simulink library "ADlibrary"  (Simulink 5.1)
undefined symbols (not defined in the file or in its folder): fifo_length, MCLK
libraries: xbsIndex_r3 x112, ADlibrary x9, xrbsControl_r3 x3

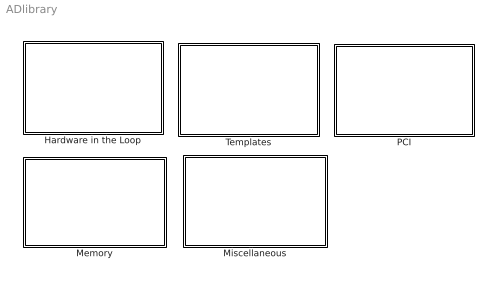
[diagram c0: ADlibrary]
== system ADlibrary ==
  Hardware in the Loop : Subsystem
  Memory : Subsystem
  Miscellaneous : Subsystem
  PCI : Subsystem
  Templates : Subsystem

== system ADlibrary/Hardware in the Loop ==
  ADMXRC DWSR IO : S-Function  AncestorBlock=ADlibrary/ADMXRC SWDR I//O  FunctionName=ADMXRCdwsr  Parameters=filename clock_freq mclk_freq input_width output_width index  mask(ADMXRC DWSR I/O){filename=, clock_freq=50, mclk_freq=, input_width=1, output_width=1, index=0}
      mask prompts: clock_freq "L Clock Frequency (MHz)"; mclk_freq "M Clock Frequency (MHz) (x2 for XRC-II)"; input_width "Width of input vector"; output_width "Width of output vector"; index "Card Index"
      mask help: Hardware in the loop block for Demand Mode DMA Write, Slave mode Read I/O with ADM-XRC/ADM-XRC II Cards.
      mask init:
      | try
      | card=admxrc_init([],index);
      | [id,sn,bt,ft]=admxrc_getinfo(card);
      | admxrc_close(card);
      | infostr=['Board Type: ' bt ' - FPGA : ' ft];
      | catch
      | infostr='No Card Detected';
      | end
      | 
      | pos=get_param(gcb,'Position');
      | width=pos(3)-pos(1);
      | height=pos(4)-pos(2);
      | if (input_width>0),istr=['Input [' num2str(input_width) ']'];else,istr='';end
      | if (output_width>0), ostr=['Output [' num2str(output_width) ']'];else,ostr='';end
      | as=get_param(gcb,'MaskIconUnits');
      | if (as(1)=='p')
      | 	im=imread('adbutton.jpg');s=get_param(gcb,'MaskDisplay');
      |     add_ad_icon(70,15);
      | else	
      | 	rm_ad_icon
      | end
  ADMXRC MMAP IO : S-Function  FunctionName=ADMXRCmmap  Parameters=filename clock_freq mclk_freq index  mask(ADMXRC MMAP I/O){filename=, clock_freq=50, mclk_freq=25, index=0}
      mask prompts: clock_freq "L Clock Frequency (MHz)"; mclk_freq "M Clock Frequency (MHz) (x2 for XRC-II)"; index "Card Index"
      mask help: Hardware in the loop block for Memory Mapped I/O Communication with ADM-XRC/ADM-XRC II Cards.
      mask init:
      | try
      | card=admxrc_init([],index);
      | [id,sn,bt,ft]=admxrc_getinfo(card);
      | admxrc_close(card);
      | infostr=['Board: ' bt ' - FPGA : ' ft];
      | catch
      | infostr='No Card Detected';
      | end
      | 
      | pos=get_param(gcb,'Position');
      | width=pos(3)-pos(1);
      | height=pos(4)-pos(2);
      | as=get_param(gcb,'MaskIconUnits');
      | if (as(1)=='p')
      | 	im=imread('adbutton.jpg');s=get_param(gcb,'MaskDisplay');
      |     add_ad_icon(70,15);
      | else	
      | 	rm_ad_icon
      | end
  ADMXRC SWDR IO : S-Function  AncestorBlock=ADlibrary/ADMXRC Slave I//O  FunctionName=ADMXRCswdr  Parameters=filename clock_freq mclk_freq input_width output_width index  mask(ADMXRC SWDR I/O){filename=, clock_freq=50, mclk_freq=, input_width=1, output_width=1, index=0}
      mask prompts: clock_freq "L Clock Frequency (MHz)"; mclk_freq "M Clock Frequency (MHz) (x2 for XRC-II)"; input_width "Width of input vector"; output_width "Width of output vector"; index "Card Index"
      mask help: Hardware in the loop block for Slave Mode Write, Demand Mode DMA Read to ADM-XRC/ADM-XRC II Cards.
      mask init:
      | try
      | card=admxrc_init([],index);
      | [id,sn,bt,ft]=admxrc_getinfo(card);
      | admxrc_close(card);
      | infostr=['Board Type: ' bt ' - FPGA : ' ft];
      | catch
      | infostr='No Card Detected';
      | end
      | 
      | pos=get_param(gcb,'Position');
      | width=pos(3)-pos(1);
      | height=pos(4)-pos(2);
      | if (input_width>0),istr=['Input [' num2str(input_width) ']'];else,istr='';end
      | if (output_width>0), ostr=['Output [' num2str(output_width) ']'];else,ostr='';end
      | as=get_param(gcb,'MaskIconUnits');
      | if (as(1)=='p')
      | 	im=imread('adbutton.jpg');s=get_param(gcb,'MaskDisplay');
      |     add_ad_icon(70,15);
      | else	
      | 	rm_ad_icon
      | end
  ADMXRC Slave IO : S-Function  AncestorBlock=ADlibrary/ADMXRC Simple I//O  FunctionName=ADMXRCslave  Parameters=filename clock_freq input_width output_width tll index  mask(ADMXRC Slave I/O){filename=, clock_freq=50, input_width=1, output_width=1, tll=1000, index=0}
      mask prompts: clock_freq "L Clock Frequency (MHz)"; input_width "Width of input vector"; output_width "Width of output vector"; tll "Terminate Loop Limit"; index "Card Index"
      mask help: Hardware in the loop block for Slave Mode Access to ADM-XRC/ADM-XRC II Cards.
      mask init:
      | try
      | card=admxrc_init([],index);
      | [id,sn,bt,ft]=admxrc_getinfo(card);
      | admxrc_close(card);
      | infostr=['Board Type: ' bt ' - FPGA : ' ft];
      | catch
      | infostr='No Card Detected';
      | end
      | 
      | pos=get_param(gcb,'Position');
      | width=pos(3)-pos(1);
      | height=pos(4)-pos(2);
      | if (input_width>0),istr=['Input [' num2str(input_width) ']'];else,istr='';end
      | if (output_width>0), ostr=['Output [' num2str(output_width) ']'];else,ostr='';end
      | as=get_param(gcb,'MaskIconUnits');
      | if (as(1)=='p')
      | 	im=imread('adbutton.jpg');s=get_param(gcb,'MaskDisplay');
      |     add_ad_icon(70,15);
      | else	
      | 	rm_ad_icon
      | end

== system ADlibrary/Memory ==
  XRCSRAM0 : Subsystem
  XRCSRAM1 : Subsystem  AncestorBlock=ADlibrary/SRAM0
  XRCSRAM2 : Subsystem  AncestorBlock=ADlibrary/SRAM0
  XRCSRAM3 : Subsystem  AncestorBlock=ADlibrary/SRAM0
  XRCSRAM4 : Subsystem  AncestorBlock=ADlibrary/SRAM0
  XRCSRAM5 : Subsystem  AncestorBlock=ADlibrary/SRAM0
  XRCSRAM7 : Subsystem

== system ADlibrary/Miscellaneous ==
  ADMXRC Board  Implementation : Subsystem  mask(Board Implementation){board=<empty>, run_synth=off, make_clean=off, userdefmods=, custom_template_file=, lvds_io_std=3.3v, clock_source=MCLK, mclk_pin=}
      mask prompts: run_synth "Run Synthesis"; make_clean "Make Clean"; userdefmods "User Defined I/O Modules"; custom_template_file "Custom Template File"; lvds_io_std "LVDS I/O Standard"; clock_source "Clock Source"; mclk_pin "MCLK Pin"
      mask help: This block allows the implementation of the system on an FPGA situated on an XRC board. This modifies the system generator VHDL and adds extra code to connect to the PCI bus, and support the ZBT SRAM and XRC I/O ports. The block can also autorun Xilinx and Third Party Synthesis tools.
      mask init:
      | as=get_param(gcb,'MaskIconUnits');
      | if (as(1)=='p')
      | 	im=imread('adbutton.jpg');s=get_param(gcb,'MaskDisplay');
      |     add_ad_icon(14,3);
      | else	
      | 	rm_ad_icon
      | end
  Complex  to int32 : S-Function  FunctionName=cplxtoint32
  HEX Constant : Subsystem  mask(HEX Constant){value=1234}
      mask prompts: value "HEX Constant"
      mask help: Hexadecimal constant
  HEX Display : S-Function  FunctionName=hexdisplay
  XRC Scope : Subsystem
  int32 to Complex : S-Function  FunctionName=int32tocplx

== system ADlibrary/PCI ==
  DWSR XRCPCI : Subsystem  AncestorBlock=ADlibrary/PCI/Slave XRCPCI  mask{no_inputs=1, no_outputs=1, circuit_lag=1, decode_delay=0}
      mask prompts: no_inputs "Number of Inputs"; no_outputs "Number of Outputs"; circuit_lag "Circuit Lag"; decode_delay "Decode Delay"
      mask init:
      | pos=get_param(gcb,'Position');
      | width=pos(3)-pos(1);height=pos(4)-pos(2);
      | if (no_inputs>0),istr=['Input [' num2str(no_inputs) ']'];else,istr='';end
      | if (no_outputs>0), ostr=['Output [' num2str(no_outputs) ']'];else,ostr='';end
      | as=get_param(gcb,'MaskIconUnits');
      | if (as(1)=='p')
      | 	im=imread('adbutton.jpg');s=get_param(gcb,'MaskDisplay');
      |     add_ad_icon(60,80);
      | else	
      | 	rm_ad_icon
      | end
  MMAP XRCPCI : Subsystem  AncestorBlock=ADlibrary/PCI/DWSR XRCPCI  mask(MMAP XRCPCI){qv132678sdfs=0}
      mask prompts: qv132678sdfs "a"
      mask init:
      | pos=get_param(gcb,'Position');
      | width=pos(3)-pos(1);height=pos(4)-pos(2);
      | as=get_param(gcb,'MaskIconUnits');
      | if (as(1)=='p')
      | 	im=imread('adbutton.jpg');s=get_param(gcb,'MaskDisplay');
      |     add_ad_icon(60,80);
      | else	
      | 	rm_ad_icon
      | end
  SWDR XRCPCI : Subsystem  AncestorBlock=ADlibrary/PCI/ADMA XRCPCI  mask{no_inputs=1, no_outputs=1, circuit_lag=4, fifo_length=256, debug=0}
      mask prompts: no_inputs "Number of Inputs"; no_outputs "Number of Outputs"; circuit_lag "Circuit Lag"; fifo_length "FIFO Length"; debug "Debug Flag"
      mask init:
      | pos=get_param(gcb,'Position');
      | width=pos(3)-pos(1);height=pos(4)-pos(2);
      | if (no_inputs>0),istr=['Input [' num2str(no_inputs) ']'];else,istr='';end
      | if (no_outputs>0), ostr=['Output [' num2str(no_outputs) ']'];else,ostr='';end
      | as=get_param(gcb,'MaskIconUnits');
      | if (as(1)=='p')
      | 	im=imread('adbutton.jpg');s=get_param(gcb,'MaskDisplay');
      |     add_ad_icon(60,80);
      | else	
      | 	rm_ad_icon
      | end
  Slave XRCPCI : Subsystem  mask{no_inputs=1, no_outputs=1, circuit_lag=1, decode_delay=0}
      mask prompts: no_inputs "Number of Inputs"; no_outputs "Number of Outputs"; circuit_lag "Circuit Lag"; decode_delay "Decode Delay"
      mask init:
      | pos=get_param(gcb,'Position');
      | width=pos(3)-pos(1);height=pos(4)-pos(2);
      | if (no_inputs>0),istr=['Input [' num2str(no_inputs) ']'];else,istr='';end
      | if (no_outputs>0), ostr=['Output [' num2str(no_outputs) ']'];else,ostr='';end
      | as=get_param(gcb,'MaskIconUnits');
      | if (as(1)=='p')
      | 	im=imread('adbutton.jpg');s=get_param(gcb,'MaskDisplay');
      |     add_ad_icon(60,80);
      | else	
      | 	rm_ad_icon
      | end

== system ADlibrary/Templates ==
  DWSR IO : Subsystem
  MMAP IO : Subsystem  AncestorBlock=ADlibrary/Templates/DWSR IO
  SWDR IO : Subsystem
  SlaveIO : Subsystem

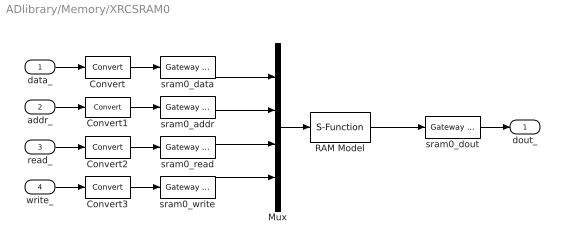
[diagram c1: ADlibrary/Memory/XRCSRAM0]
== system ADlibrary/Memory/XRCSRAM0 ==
  data_ : Inport
  addr_ : Inport  Port=2
  read_ : Inport  Port=3
  write_ : Inport  Port=4
  Convert : xbsIndex_r3/Convert  arith_type="Signed  (2's comp)"  n_bits=32  bin_pt=0  quantization=Truncate  overflow=Wrap  latency=0  explicit_period=off  period=1  dbl_ovrd=off  inserted_by_tool=off
  Convert1 : xbsIndex_r3/Convert  arith_type=Unsigned  n_bits=20  bin_pt=0  quantization=Truncate  overflow=Wrap  latency=0  explicit_period=off  period=1  dbl_ovrd=off  inserted_by_tool=off
  Convert2 : xbsIndex_r3/Convert  arith_type=Boolean  n_bits=1  bin_pt=0  quantization=Truncate  overflow=Wrap  latency=0  explicit_period=off  period=1  dbl_ovrd=off  inserted_by_tool=off
  Convert3 : xbsIndex_r3/Convert  arith_type=Boolean  n_bits=1  bin_pt=0  quantization=Truncate  overflow=Wrap  latency=0  explicit_period=off  period=1  dbl_ovrd=off  inserted_by_tool=off
  Mux : Mux
  RAM Model : S-Function  FunctionName=modelram  Parameters=0
  sram0_addr : xbsIndex_r3/Gateway Out  hdl_port=on  timing_constraint=None  locs_specified=off  LOCs={}  needs_fixed_name=on
  sram0_data : xbsIndex_r3/Gateway Out  hdl_port=on  timing_constraint=None  locs_specified=off  LOCs={}  needs_fixed_name=on
  sram0_dout : xbsIndex_r3/Gateway In  arith_type="Signed  (2's comp)"  n_bits=32  bin_pt=0  quantization=Truncate  overflow=Wrap  period=1  timing_constraint=None  locs_specified=off  LOCs={}  needs_fixed_name=on  dbl_ovrd=off
  sram0_read : xbsIndex_r3/Gateway Out  hdl_port=on  timing_constraint=None  locs_specified=off  LOCs={}  needs_fixed_name=on
  sram0_write : xbsIndex_r3/Gateway Out  hdl_port=on  timing_constraint=None  locs_specified=off  LOCs={}  needs_fixed_name=on
  dout_ : Outport
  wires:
  data_/1 -> Convert/1
  addr_/1 -> Convert1/1
  read_/1 -> Convert2/1
  sram0_dout/1 -> dout_/1
  Convert/1 -> sram0_data/1
  Convert1/1 -> sram0_addr/1
  Convert2/1 -> sram0_read/1
  RAM Model/1 -> sram0_dout/1
  Mux/1 -> RAM Model/1
  sram0_data/1 -> Mux/1
  sram0_addr/1 -> Mux/2
  sram0_read/1 -> Mux/3
  write_/1 -> Convert3/1
  Convert3/1 -> sram0_write/1
  sram0_write/1 -> Mux/4

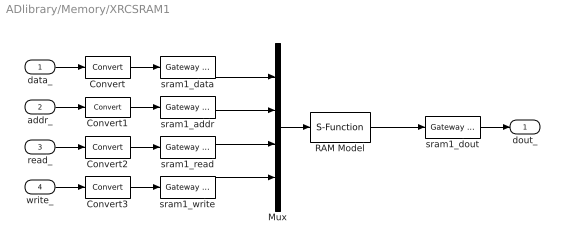
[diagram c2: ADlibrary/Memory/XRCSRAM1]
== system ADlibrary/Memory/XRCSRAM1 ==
  data_ : Inport
  addr_ : Inport  Port=2
  read_ : Inport  Port=3
  write_ : Inport  Port=4
  Convert : xbsIndex_r3/Convert  arith_type="Signed  (2's comp)"  n_bits=32  bin_pt=0  quantization=Truncate  overflow=Wrap  latency=0  explicit_period=off  period=1  dbl_ovrd=off  inserted_by_tool=off
  Convert1 : xbsIndex_r3/Convert  arith_type=Unsigned  n_bits=20  bin_pt=0  quantization=Truncate  overflow=Wrap  latency=0  explicit_period=off  period=1  dbl_ovrd=off  inserted_by_tool=off
  Convert2 : xbsIndex_r3/Convert  arith_type=Boolean  n_bits=1  bin_pt=0  quantization=Truncate  overflow=Wrap  latency=0  explicit_period=off  period=1  dbl_ovrd=off  inserted_by_tool=off
  Convert3 : xbsIndex_r3/Convert  arith_type=Boolean  n_bits=1  bin_pt=0  quantization=Truncate  overflow=Wrap  latency=0  explicit_period=off  period=1  dbl_ovrd=off  inserted_by_tool=off
  Mux : Mux
  RAM Model : S-Function  FunctionName=modelram  Parameters=1
  sram1_addr : xbsIndex_r3/Gateway Out  hdl_port=on  timing_constraint=None  locs_specified=off  LOCs={}  needs_fixed_name=on
  sram1_data : xbsIndex_r3/Gateway Out  hdl_port=on  timing_constraint=None  locs_specified=off  LOCs={}  needs_fixed_name=on
  sram1_dout : xbsIndex_r3/Gateway In  arith_type="Signed  (2's comp)"  n_bits=32  bin_pt=0  quantization=Truncate  overflow=Wrap  period=1  timing_constraint=None  locs_specified=off  LOCs={}  needs_fixed_name=on  dbl_ovrd=off
  sram1_read : xbsIndex_r3/Gateway Out  hdl_port=on  timing_constraint=None  locs_specified=off  LOCs={}  needs_fixed_name=on
  sram1_write : xbsIndex_r3/Gateway Out  hdl_port=on  timing_constraint=None  locs_specified=off  LOCs={}  needs_fixed_name=on
  dout_ : Outport
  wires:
  sram1_write/1 -> Mux/4
  Convert3/1 -> sram1_write/1
  write_/1 -> Convert3/1
  sram1_read/1 -> Mux/3
  sram1_addr/1 -> Mux/2
  sram1_data/1 -> Mux/1
  Mux/1 -> RAM Model/1
  RAM Model/1 -> sram1_dout/1
  Convert2/1 -> sram1_read/1
  Convert1/1 -> sram1_addr/1
  Convert/1 -> sram1_data/1
  sram1_dout/1 -> dout_/1
  read_/1 -> Convert2/1
  addr_/1 -> Convert1/1
  data_/1 -> Convert/1

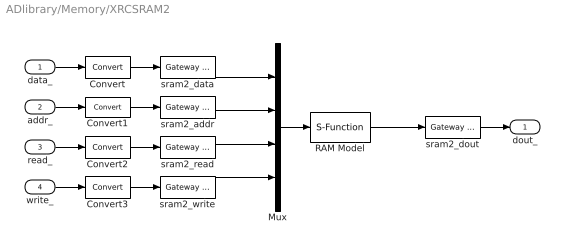
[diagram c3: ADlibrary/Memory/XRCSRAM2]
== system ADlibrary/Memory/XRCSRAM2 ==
  data_ : Inport
  addr_ : Inport  Port=2
  read_ : Inport  Port=3
  write_ : Inport  Port=4
  Convert : xbsIndex_r3/Convert  arith_type="Signed  (2's comp)"  n_bits=32  bin_pt=0  quantization=Truncate  overflow=Wrap  latency=0  explicit_period=off  period=1  dbl_ovrd=off  inserted_by_tool=off
  Convert1 : xbsIndex_r3/Convert  arith_type=Unsigned  n_bits=20  bin_pt=0  quantization=Truncate  overflow=Wrap  latency=0  explicit_period=off  period=1  dbl_ovrd=off  inserted_by_tool=off
  Convert2 : xbsIndex_r3/Convert  arith_type=Boolean  n_bits=1  bin_pt=0  quantization=Truncate  overflow=Wrap  latency=0  explicit_period=off  period=1  dbl_ovrd=off  inserted_by_tool=off
  Convert3 : xbsIndex_r3/Convert  arith_type=Boolean  n_bits=1  bin_pt=0  quantization=Truncate  overflow=Wrap  latency=0  explicit_period=off  period=1  dbl_ovrd=off  inserted_by_tool=off
  Mux : Mux
  RAM Model : S-Function  FunctionName=modelram  Parameters=2
  sram2_addr : xbsIndex_r3/Gateway Out  hdl_port=on  timing_constraint=None  locs_specified=off  LOCs={}  needs_fixed_name=on
  sram2_data : xbsIndex_r3/Gateway Out  hdl_port=on  timing_constraint=None  locs_specified=off  LOCs={}  needs_fixed_name=on
  sram2_dout : xbsIndex_r3/Gateway In  arith_type="Signed  (2's comp)"  n_bits=32  bin_pt=0  quantization=Truncate  overflow=Wrap  period=1  timing_constraint=None  locs_specified=off  LOCs={}  needs_fixed_name=on  dbl_ovrd=off
  sram2_read : xbsIndex_r3/Gateway Out  hdl_port=on  timing_constraint=None  locs_specified=off  LOCs={}  needs_fixed_name=on
  sram2_write : xbsIndex_r3/Gateway Out  hdl_port=on  timing_constraint=None  locs_specified=off  LOCs={}  needs_fixed_name=on
  dout_ : Outport
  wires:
  sram2_write/1 -> Mux/4
  Convert3/1 -> sram2_write/1
  write_/1 -> Convert3/1
  sram2_read/1 -> Mux/3
  sram2_addr/1 -> Mux/2
  sram2_data/1 -> Mux/1
  Mux/1 -> RAM Model/1
  RAM Model/1 -> sram2_dout/1
  Convert2/1 -> sram2_read/1
  Convert1/1 -> sram2_addr/1
  Convert/1 -> sram2_data/1
  sram2_dout/1 -> dout_/1
  read_/1 -> Convert2/1
  addr_/1 -> Convert1/1
  data_/1 -> Convert/1

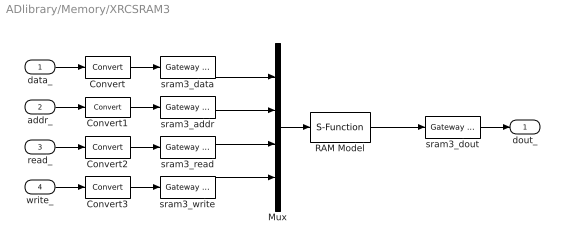
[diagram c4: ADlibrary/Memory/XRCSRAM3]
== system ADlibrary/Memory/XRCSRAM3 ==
  data_ : Inport
  addr_ : Inport  Port=2
  read_ : Inport  Port=3
  write_ : Inport  Port=4
  Convert : xbsIndex_r3/Convert  arith_type="Signed  (2's comp)"  n_bits=32  bin_pt=0  quantization=Truncate  overflow=Wrap  latency=0  explicit_period=off  period=1  dbl_ovrd=off  inserted_by_tool=off
  Convert1 : xbsIndex_r3/Convert  arith_type=Unsigned  n_bits=20  bin_pt=0  quantization=Truncate  overflow=Wrap  latency=0  explicit_period=off  period=1  dbl_ovrd=off  inserted_by_tool=off
  Convert2 : xbsIndex_r3/Convert  arith_type=Boolean  n_bits=1  bin_pt=0  quantization=Truncate  overflow=Wrap  latency=0  explicit_period=off  period=1  dbl_ovrd=off  inserted_by_tool=off
  Convert3 : xbsIndex_r3/Convert  arith_type=Boolean  n_bits=1  bin_pt=0  quantization=Truncate  overflow=Wrap  latency=0  explicit_period=off  period=1  dbl_ovrd=off  inserted_by_tool=off
  Mux : Mux
  RAM Model : S-Function  FunctionName=modelram  Parameters=3
  sram3_addr : xbsIndex_r3/Gateway Out  hdl_port=on  timing_constraint=None  locs_specified=off  LOCs={}  needs_fixed_name=on
  sram3_data : xbsIndex_r3/Gateway Out  hdl_port=on  timing_constraint=None  locs_specified=off  LOCs={}  needs_fixed_name=on
  sram3_dout : xbsIndex_r3/Gateway In  arith_type="Signed  (2's comp)"  n_bits=32  bin_pt=0  quantization=Truncate  overflow=Wrap  period=1  timing_constraint=None  locs_specified=off  LOCs={}  needs_fixed_name=on  dbl_ovrd=off
  sram3_read : xbsIndex_r3/Gateway Out  hdl_port=on  timing_constraint=None  locs_specified=off  LOCs={}  needs_fixed_name=on
  sram3_write : xbsIndex_r3/Gateway Out  hdl_port=on  timing_constraint=None  locs_specified=off  LOCs={}  needs_fixed_name=on
  dout_ : Outport
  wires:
  sram3_write/1 -> Mux/4
  Convert3/1 -> sram3_write/1
  write_/1 -> Convert3/1
  sram3_read/1 -> Mux/3
  sram3_addr/1 -> Mux/2
  sram3_data/1 -> Mux/1
  Mux/1 -> RAM Model/1
  RAM Model/1 -> sram3_dout/1
  Convert2/1 -> sram3_read/1
  Convert1/1 -> sram3_addr/1
  Convert/1 -> sram3_data/1
  sram3_dout/1 -> dout_/1
  read_/1 -> Convert2/1
  addr_/1 -> Convert1/1
  data_/1 -> Convert/1

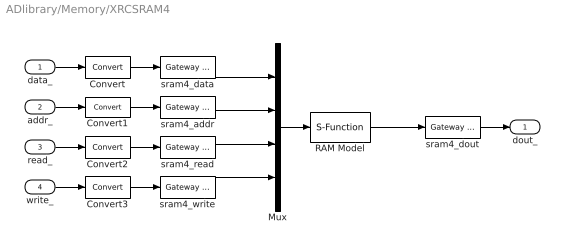
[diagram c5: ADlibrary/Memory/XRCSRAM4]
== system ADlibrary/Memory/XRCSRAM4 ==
  data_ : Inport
  addr_ : Inport  Port=2
  read_ : Inport  Port=3
  write_ : Inport  Port=4
  Convert : xbsIndex_r3/Convert  arith_type="Signed  (2's comp)"  n_bits=32  bin_pt=0  quantization=Truncate  overflow=Wrap  latency=0  explicit_period=off  period=1  dbl_ovrd=off  inserted_by_tool=off
  Convert1 : xbsIndex_r3/Convert  arith_type=Unsigned  n_bits=20  bin_pt=0  quantization=Truncate  overflow=Wrap  latency=0  explicit_period=off  period=1  dbl_ovrd=off  inserted_by_tool=off
  Convert2 : xbsIndex_r3/Convert  arith_type=Boolean  n_bits=1  bin_pt=0  quantization=Truncate  overflow=Wrap  latency=0  explicit_period=off  period=1  dbl_ovrd=off  inserted_by_tool=off
  Convert3 : xbsIndex_r3/Convert  arith_type=Boolean  n_bits=1  bin_pt=0  quantization=Truncate  overflow=Wrap  latency=0  explicit_period=off  period=1  dbl_ovrd=off  inserted_by_tool=off
  Mux : Mux
  RAM Model : S-Function  FunctionName=modelram  Parameters=4
  sram4_addr : xbsIndex_r3/Gateway Out  hdl_port=on  timing_constraint=None  locs_specified=off  LOCs={}  needs_fixed_name=on
  sram4_data : xbsIndex_r3/Gateway Out  hdl_port=on  timing_constraint=None  locs_specified=off  LOCs={}  needs_fixed_name=on
  sram4_dout : xbsIndex_r3/Gateway In  arith_type="Signed  (2's comp)"  n_bits=32  bin_pt=0  quantization=Truncate  overflow=Wrap  period=1  timing_constraint=None  locs_specified=off  LOCs={}  needs_fixed_name=on  dbl_ovrd=off
  sram4_read : xbsIndex_r3/Gateway Out  hdl_port=on  timing_constraint=None  locs_specified=off  LOCs={}  needs_fixed_name=on
  sram4_write : xbsIndex_r3/Gateway Out  hdl_port=on  timing_constraint=None  locs_specified=off  LOCs={}  needs_fixed_name=on
  dout_ : Outport
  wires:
  data_/1 -> Convert/1
  addr_/1 -> Convert1/1
  read_/1 -> Convert2/1
  sram4_dout/1 -> dout_/1
  Convert/1 -> sram4_data/1
  Convert1/1 -> sram4_addr/1
  Convert2/1 -> sram4_read/1
  RAM Model/1 -> sram4_dout/1
  Mux/1 -> RAM Model/1
  sram4_data/1 -> Mux/1
  sram4_addr/1 -> Mux/2
  sram4_read/1 -> Mux/3
  write_/1 -> Convert3/1
  Convert3/1 -> sram4_write/1
  sram4_write/1 -> Mux/4

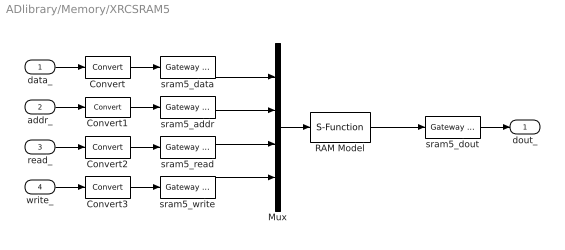
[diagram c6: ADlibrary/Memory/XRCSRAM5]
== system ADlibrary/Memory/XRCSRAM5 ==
  data_ : Inport
  addr_ : Inport  Port=2
  read_ : Inport  Port=3
  write_ : Inport  Port=4
  Convert : xbsIndex_r3/Convert  arith_type="Signed  (2's comp)"  n_bits=32  bin_pt=0  quantization=Truncate  overflow=Wrap  latency=0  explicit_period=off  period=1  dbl_ovrd=off  inserted_by_tool=off
  Convert1 : xbsIndex_r3/Convert  arith_type=Unsigned  n_bits=20  bin_pt=0  quantization=Truncate  overflow=Wrap  latency=0  explicit_period=off  period=1  dbl_ovrd=off  inserted_by_tool=off
  Convert2 : xbsIndex_r3/Convert  arith_type=Boolean  n_bits=1  bin_pt=0  quantization=Truncate  overflow=Wrap  latency=0  explicit_period=off  period=1  dbl_ovrd=off  inserted_by_tool=off
  Convert3 : xbsIndex_r3/Convert  arith_type=Boolean  n_bits=1  bin_pt=0  quantization=Truncate  overflow=Wrap  latency=0  explicit_period=off  period=1  dbl_ovrd=off  inserted_by_tool=off
  Mux : Mux
  RAM Model : S-Function  FunctionName=modelram  Parameters=5
  sram5_addr : xbsIndex_r3/Gateway Out  hdl_port=on  timing_constraint=None  locs_specified=off  LOCs={}  needs_fixed_name=on
  sram5_data : xbsIndex_r3/Gateway Out  hdl_port=on  timing_constraint=None  locs_specified=off  LOCs={}  needs_fixed_name=on
  sram5_dout : xbsIndex_r3/Gateway In  arith_type="Signed  (2's comp)"  n_bits=32  bin_pt=0  quantization=Truncate  overflow=Wrap  period=1  timing_constraint=None  locs_specified=off  LOCs={}  needs_fixed_name=on  dbl_ovrd=off
  sram5_read : xbsIndex_r3/Gateway Out  hdl_port=on  timing_constraint=None  locs_specified=off  LOCs={}  needs_fixed_name=on
  sram5_write : xbsIndex_r3/Gateway Out  hdl_port=on  timing_constraint=None  locs_specified=off  LOCs={}  needs_fixed_name=on
  dout_ : Outport
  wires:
  data_/1 -> Convert/1
  addr_/1 -> Convert1/1
  read_/1 -> Convert2/1
  sram5_dout/1 -> dout_/1
  Convert/1 -> sram5_data/1
  Convert1/1 -> sram5_addr/1
  Convert2/1 -> sram5_read/1
  RAM Model/1 -> sram5_dout/1
  Mux/1 -> RAM Model/1
  sram5_data/1 -> Mux/1
  sram5_addr/1 -> Mux/2
  sram5_read/1 -> Mux/3
  write_/1 -> Convert3/1
  Convert3/1 -> sram5_write/1
  sram5_write/1 -> Mux/4

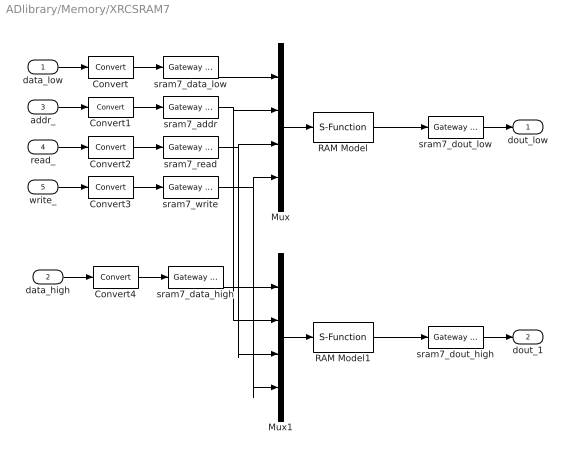
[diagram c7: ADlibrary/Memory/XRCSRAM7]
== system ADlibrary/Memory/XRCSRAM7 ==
  data_low : Inport
  data_high : Inport  Port=2
  addr_ : Inport  Port=3
  read_ : Inport  Port=4
  write_ : Inport  Port=5
  Convert : xbsIndex_r3/Convert  arith_type="Signed  (2's comp)"  n_bits=32  bin_pt=0  quantization=Truncate  overflow=Wrap  latency=0  explicit_period=off  period=1  dbl_ovrd=off  inserted_by_tool=off
  Convert1 : xbsIndex_r3/Convert  arith_type=Unsigned  n_bits=20  bin_pt=0  quantization=Truncate  overflow=Wrap  latency=0  explicit_period=off  period=1  dbl_ovrd=off  inserted_by_tool=off
  Convert2 : xbsIndex_r3/Convert  arith_type=Boolean  n_bits=1  bin_pt=0  quantization=Truncate  overflow=Wrap  latency=0  explicit_period=off  period=1  dbl_ovrd=off  inserted_by_tool=off
  Convert3 : xbsIndex_r3/Convert  arith_type=Boolean  n_bits=1  bin_pt=0  quantization=Truncate  overflow=Wrap  latency=0  explicit_period=off  period=1  dbl_ovrd=off  inserted_by_tool=off
  Convert4 : xbsIndex_r3/Convert  arith_type="Signed  (2's comp)"  n_bits=32  bin_pt=0  quantization=Truncate  overflow=Wrap  latency=0  explicit_period=off  period=1  dbl_ovrd=off  inserted_by_tool=off
  Mux : Mux
  Mux1 : Mux
  RAM Model : S-Function  FunctionName=modelram  Parameters=0
  RAM Model1 : S-Function  FunctionName=modelram  Parameters=1
  sram7_addr : xbsIndex_r3/Gateway Out  hdl_port=on  timing_constraint=None  locs_specified=off  LOCs={}  needs_fixed_name=on
  sram7_data_high : xbsIndex_r3/Gateway Out  hdl_port=on  timing_constraint=None  locs_specified=off  LOCs={}  needs_fixed_name=on
  sram7_data_low : xbsIndex_r3/Gateway Out  hdl_port=on  timing_constraint=None  locs_specified=off  LOCs={}  needs_fixed_name=on
  sram7_dout_high : xbsIndex_r3/Gateway In  arith_type="Signed  (2's comp)"  n_bits=32  bin_pt=0  quantization=Truncate  overflow=Wrap  period=1  timing_constraint=None  locs_specified=off  LOCs={}  needs_fixed_name=on  dbl_ovrd=off
  sram7_dout_low : xbsIndex_r3/Gateway In  arith_type="Signed  (2's comp)"  n_bits=32  bin_pt=0  quantization=Truncate  overflow=Wrap  period=1  timing_constraint=None  locs_specified=off  LOCs={}  needs_fixed_name=on  dbl_ovrd=off
  sram7_read : xbsIndex_r3/Gateway Out  hdl_port=on  timing_constraint=None  locs_specified=off  LOCs={}  needs_fixed_name=on
  sram7_write : xbsIndex_r3/Gateway Out  hdl_port=on  timing_constraint=None  locs_specified=off  LOCs={}  needs_fixed_name=on
  dout_low : Outport
  dout_1 : Outport  Port=2
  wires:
  data_low/1 -> Convert/1
  addr_/1 -> Convert1/1
  read_/1 -> Convert2/1
  sram7_dout_low/1 -> dout_low/1
  Convert/1 -> sram7_data_low/1
  Convert1/1 -> sram7_addr/1
  Convert2/1 -> sram7_read/1
  RAM Model/1 -> sram7_dout_low/1
  Mux/1 -> RAM Model/1
  sram7_data_low/1 -> Mux/1
  sram7_addr/1 -> Mux/2, Mux1/2
  sram7_read/1 -> Mux/3, Mux1/3
  write_/1 -> Convert3/1
  Convert3/1 -> sram7_write/1
  sram7_write/1 -> Mux/4, Mux1/4
  data_high/1 -> Convert4/1
  Convert4/1 -> sram7_data_high/1
  sram7_data_high/1 -> Mux1/1
  sram7_dout_high/1 -> dout_1/1
  RAM Model1/1 -> sram7_dout_high/1
  Mux1/1 -> RAM Model1/1

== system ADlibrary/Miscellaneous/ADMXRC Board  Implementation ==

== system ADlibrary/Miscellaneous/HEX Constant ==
  Data Type Conversion : DataTypeConversion  DataType=uint32
  Hex Constant : S-Function  FunctionName=hexconstant  Parameters=value
  Out1 : Outport
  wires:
  Data Type Conversion/1 -> Out1/1
  Hex Constant/1 -> Data Type Conversion/1

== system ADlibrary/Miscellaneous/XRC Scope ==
  Data : Inport
  Trigger : Inport  Port=2
  Addr  Counter [7:0] : xrbsControl_r3/Moore State Machine  next_state_matrix=[0 1;1 2;2 3;3 4;4 5;5 6;6 7;7 8;8 9;9 10;10 11;11 12;12 13;13 14;14 15;15 16;16 17;17 18;18 19;19 20;20 21;21 22;22 23;23 24;24 25;25 26;26 27;27 28;28 29;29 30;30 31;31 32;32 33;33 34;34 35;35 36;36 37;37 38;38 39;39 40;40 41;41 42;42 43;43 44;44 45;45 46;46 47;47 48;48 49;49 50;50 51;51 52;52 53;53 54;54 55;55 56;56 57;57 58;58 59;59 60;60 61;61 62;62 63;63 64;64 65;65 66;66 67;67 68;68 69;69 7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  output_matrix=[0;0;0;0;0;0;0;0;0;0;0;0;0;0;0;0;0;0;0;0;0;0;0;0;0;0;0;0;0;0;0;0;0;0;0;0;0;0;0;0;0;0;0;0;0;0;0;0;0;0;0;0;0;0;0;0;0;0;0;0;0;0;0;0;0;0;0;0;0;0;0;0;0;0;0;0;0;0;0;0;0;0;0;0;0;0;0;0;0;0;0;0;0;0;0;0;0;0;0;0;0;0;0;0;0;0;0;0;0;0;0;0;0;0;0;0;0;0;0;0;0;0;0;0;0;0;0;0;0;0;0;0;0;0;0;0;0;0;0;0;0;0;0;0;0;0;0;0;0;0;0;0;0;0;0;0;0;0;0;0;0;0;0;0;0;0;0;0;0;0;0;0;0;0;0;0;0;0;0;0;0;0;0;0;0;0;0;0;0;0;0;0;0;0;0;0;0;0;0;0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  n_bits=1  period=1
  Addr Counter [15:8] : xrbsControl_r3/Moore State Machine  next_state_matrix=[0 1;1 2;2 3;3 4;4 5;5 6;6 7;7 8;8 9;9 10;10 11;11 12;12 13;13 14;14 15;15 16;16 17;17 18;18 19;19 20;20 21;21 22;22 23;23 24;24 25;25 26;26 27;27 28;28 29;29 30;30 31;31 32;32 33;33 34;34 35;35 36;36 37;37 38;38 39;39 40;40 41;41 42;42 43;43 44;44 45;45 46;46 47;47 48;48 49;49 50;50 51;51 52;52 53;53 54;54 55;55 56;56 57;57 58;58 59;59 60;60 61;61 62;62 63;63 64;64 65;65 66;66 67;67 68;68 69;69 7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  output_matrix=[0;0;0;0;0;0;0;0;0;0;0;0;0;0;0;0;0;0;0;0;0;0;0;0;0;0;0;0;0;0;0;0;0;0;0;0;0;0;0;0;0;0;0;0;0;0;0;0;0;0;0;0;0;0;0;0;0;0;0;0;0;0;0;0;0;0;0;0;0;0;0;0;0;0;0;0;0;0;0;0;0;0;0;0;0;0;0;0;0;0;0;0;0;0;0;0;0;0;0;0;0;0;0;0;0;0;0;0;0;0;0;0;0;0;0;0;0;0;0;0;0;0;0;0;0;0;0;0;0;0;0;0;0;0;0;0;0;0;0;0;0;0;0;0;0;0;0;0;0;0;0;0;0;0;0;0;0;0;0;0;0;0;0;0;0;0;0;0;0;0;0;0;0;0;0;0;0;0;0;0;0;0;0;0;0;0;0;0;0;0;0;0;0;0;0;0;0;0;0;0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  n_bits=1  period=1
  Concat : xbsIndex_r3/Concat  Orientation=left  explicit_period=off  period=1  dbl_ovrd=off
  Concat1 : xbsIndex_r3/Concat  explicit_period=off  period=1  dbl_ovrd=off
  Constant : xbsIndex_r3/Constant  const=0  arith_type=Unsigned  n_bits=1  bin_pt=0  explicit_period=on  period=1  dbl_ovrd=off
  Logical : xbsIndex_r3/Logical  logical_function=AND  inputs=2  precision=Full  arith_type=Unsigned  n_bits=8  bin_pt=2  align_bp=on  latency=0  explicit_period=off  period=1  en=off  dbl_ovrd=off
  Mealy State Machine : xrbsControl_r3/Mealy State Machine  next_state_matrix=[0 1 0 1; 1 1 2 2; 2 2 2 2]  output_matrix=[0 1 0 1; 1 1 0 0; 0 0 0 0]  n_bits=1  period=1
  Terminator : Terminator
  To Workspace : ToWorkspace  VariableName=XRCScopeData  SampleTime=-1  SaveFormat=Structure
  To Workspace1 : ToWorkspace  VariableName=XRCScopeState  SampleTime=-1  SaveFormat=Structure
  XRC Scope Data : xbsIndex_r3/Gateway Out  hdl_port=off  timing_constraint=None  locs_specified=off  LOCs={}  needs_fixed_name=off
  XRC Scope State : xbsIndex_r3/Gateway Out  hdl_port=off  timing_constraint=None  locs_specified=off  LOCs={}  needs_fixed_name=off
  XRCSRAM2 : ADlibrary/Memory/XRCSRAM2  AncestorBlock=ADlibrary/SRAM0
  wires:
  XRC Scope State/1 -> To Workspace1/1
  XRC Scope Data/1 -> To Workspace/1
  Mealy State Machine/1 -> XRC Scope State/1
  XRCSRAM2/1 -> Terminator/1
  Addr Counter [15:8]/2 -> Concat1/1
  Concat1/1 -> Mealy State Machine/1
  Trigger/1 -> Concat1/2
  Constant/1 -> XRCSRAM2/3
  Concat/1 -> XRCSRAM2/2
  Addr Counter [15:8]/1 -> Concat/1
  Addr  Counter [7:0]/1 -> Concat/2
  Logical/1 -> Addr Counter [15:8]/1
  Addr  Counter [7:0]/2 -> Logical/1
  Mealy State Machine/2 -> Logical/2, Addr  Counter [7:0]/1, XRCSRAM2/4
  Data/1 -> XRC Scope Data/1, XRCSRAM2/1

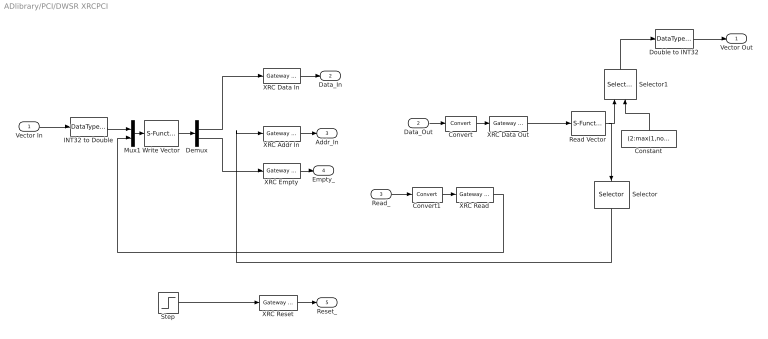
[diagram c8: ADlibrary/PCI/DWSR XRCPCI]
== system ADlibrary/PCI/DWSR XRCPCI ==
  Vector In : Inport
  Data_Out : Inport  Port=2
  Read_ : Inport  Port=3
  Constant : Constant  Orientation=up  Value=(2:max(1,no_outputs)+1)-(no_outputs==0)
  Convert : xbsIndex_r3/Convert  arith_type=Unsigned  n_bits=32  bin_pt=0  quantization=Truncate  overflow=Wrap  latency=0  explicit_period=on  period=1  dbl_ovrd=off  inserted_by_tool=off
  Convert1 : xbsIndex_r3/Convert  arith_type=Boolean  n_bits=1  bin_pt=0  quantization=Truncate  overflow=Wrap  latency=0  explicit_period=on  period=1  dbl_ovrd=off  inserted_by_tool=off
  Demux : Demux  Outputs=2
  Double to INT32 : DataTypeConversion  DataType=uint32
  INT32 to Double : DataTypeConversion  DataType=double
  Mux1 : Mux  Inputs=2
  Read Vector : S-Function  FunctionName=readvec_slave2  Parameters=no_inputs no_outputs circuit_lag decode_delay
  Selector : Selector  Orientation=down
  Selector1 : Selector  Orientation=up  ElementSrc=External
  Step : Step  Before=1  After=0  SampleTime=1
  Write Vector : S-Function  FunctionName=writevec_dma  Parameters=no_inputs no_outputs circuit_lag fifo_length
  XRC Addr In : xbsIndex_r3/Gateway In  arith_type=Unsigned  n_bits=22  bin_pt=0  quantization=Truncate  overflow=Wrap  period=1  timing_constraint=None  locs_specified=off  LOCs={}  needs_fixed_name=on  dbl_ovrd=off
  XRC Data In : xbsIndex_r3/Gateway In  arith_type=Unsigned  n_bits=32  bin_pt=0  quantization=Truncate  overflow=Wrap  period=1  timing_constraint=None  locs_specified=off  LOCs={}  needs_fixed_name=on  dbl_ovrd=off
  XRC Data Out : xbsIndex_r3/Gateway Out  hdl_port=on  timing_constraint=None  locs_specified=off  LOCs={}  needs_fixed_name=on
  XRC Empty : xbsIndex_r3/Gateway In  arith_type=Boolean  n_bits=1  bin_pt=0  quantization=Truncate  overflow=Wrap  period=1  timing_constraint=None  locs_specified=off  LOCs={}  needs_fixed_name=on  dbl_ovrd=off
  XRC Read : xbsIndex_r3/Gateway Out  hdl_port=on  timing_constraint=None  locs_specified=off  LOCs={}  needs_fixed_name=on
  XRC Reset : xbsIndex_r3/Gateway In  arith_type=Boolean  n_bits=1  bin_pt=0  quantization=Truncate  overflow=Wrap  period=1  timing_constraint=None  locs_specified=off  LOCs={}  needs_fixed_name=on  dbl_ovrd=off
  Vector Out : Outport
  Data_In : Outport  Port=2
  Addr_In : Outport  Port=3
  Empty_ : Outport  Port=4
  Reset_ : Outport  Port=5
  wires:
  XRC Read/1 -> Mux1/2
  Mux1/1 -> Write Vector/1
  INT32 to Double/1 -> Mux1/1
  Step/1 -> XRC Reset/1
  Vector In/1 -> INT32 to Double/1
  Double to INT32/1 -> Vector Out/1
  XRC Data Out/1 -> Read Vector/1
  Convert/1 -> XRC Data Out/1
  Convert1/1 -> XRC Read/1
  Data_Out/1 -> Convert/1
  Read_/1 -> Convert1/1
  XRC Data In/1 -> Data_In/1
  XRC Addr In/1 -> Addr_In/1
  XRC Empty/1 -> Empty_/1
  XRC Reset/1 -> Reset_/1
  Read Vector/1 -> Selector1/1, Selector/1
  Selector1/1 -> Double to INT32/1
  Constant/1 -> Selector1/2
  Write Vector/1 -> Demux/1
  Demux/1 -> XRC Data In/1
  Demux/2 -> XRC Empty/1
  Selector/1 -> XRC Addr In/1

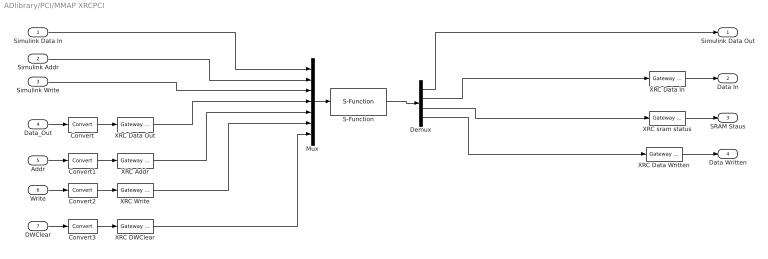
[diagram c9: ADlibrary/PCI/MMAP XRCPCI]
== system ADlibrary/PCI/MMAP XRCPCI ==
  Simulink Data In : Inport
  Simulink Addr : Inport  Port=2
  Simulink Write : Inport  Port=3
  Data_Out : Inport  Port=4
  Addr : Inport  Port=5
  Write : Inport  Port=6
  DWClear : Inport  Port=7
  Convert : xbsIndex_r3/Convert  arith_type=Unsigned  n_bits=32  bin_pt=0  quantization=Truncate  overflow=Wrap  latency=0  explicit_period=on  period=1  dbl_ovrd=off  inserted_by_tool=off
  Convert1 : xbsIndex_r3/Convert  arith_type=Unsigned  n_bits=9  bin_pt=0  quantization=Truncate  overflow=Wrap  latency=0  explicit_period=on  period=1  dbl_ovrd=off  inserted_by_tool=off
  Convert2 : xbsIndex_r3/Convert  arith_type=Boolean  n_bits=9  bin_pt=0  quantization=Truncate  overflow=Wrap  latency=0  explicit_period=on  period=1  dbl_ovrd=off  inserted_by_tool=off
  Convert3 : xbsIndex_r3/Convert  arith_type=Boolean  n_bits=9  bin_pt=0  quantization=Truncate  overflow=Wrap  latency=0  explicit_period=on  period=1  dbl_ovrd=off  inserted_by_tool=off
  Demux : Demux
  Mux : Mux  Inputs=7
  S-Function : S-Function  FunctionName=modelmmap
  XRC Addr : xbsIndex_r3/Gateway Out  hdl_port=on  timing_constraint=None  locs_specified=off  LOCs={}  needs_fixed_name=on
  XRC DWClear : xbsIndex_r3/Gateway Out  hdl_port=on  timing_constraint=None  locs_specified=off  LOCs={}  needs_fixed_name=on
  XRC Data In : xbsIndex_r3/Gateway In  arith_type=Unsigned  n_bits=32  bin_pt=0  quantization=Truncate  overflow=Wrap  period=1  timing_constraint=None  locs_specified=off  LOCs={}  needs_fixed_name=on  dbl_ovrd=off
  XRC Data Out : xbsIndex_r3/Gateway Out  hdl_port=on  timing_constraint=None  locs_specified=off  LOCs={}  needs_fixed_name=on
  XRC Data Written : xbsIndex_r3/Gateway In  arith_type=Boolean  n_bits=6  bin_pt=0  quantization=Truncate  overflow=Wrap  period=1  timing_constraint=None  locs_specified=off  LOCs={}  needs_fixed_name=on  dbl_ovrd=off
  XRC Write : xbsIndex_r3/Gateway Out  hdl_port=on  timing_constraint=None  locs_specified=off  LOCs={}  needs_fixed_name=on
  XRC sram status : xbsIndex_r3/Gateway In  arith_type=Unsigned  n_bits=6  bin_pt=0  quantization=Truncate  overflow=Wrap  period=1  timing_constraint=None  locs_specified=off  LOCs={}  needs_fixed_name=on  dbl_ovrd=off
  Simulink Data Out : Outport
  Data In : Outport  Port=2
  SRAM Staus : Outport  Port=3
  Data Written : Outport  Port=4
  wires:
  Simulink Data In/1 -> Mux/1
  Simulink Addr/1 -> Mux/2
  Simulink Write/1 -> Mux/3
  Data_Out/1 -> Convert/1
  Addr/1 -> Convert1/1
  Write/1 -> Convert2/1
  XRC Data Out/1 -> Mux/4
  XRC Addr/1 -> Mux/5
  XRC Write/1 -> Mux/6
  XRC Data In/1 -> Data In/1
  XRC sram status/1 -> SRAM Staus/1
  Convert/1 -> XRC Data Out/1
  Convert1/1 -> XRC Addr/1
  Convert2/1 -> XRC Write/1
  Demux/1 -> Simulink Data Out/1
  Demux/2 -> XRC Data In/1
  Demux/3 -> XRC sram status/1
  Mux/1 -> S-Function/1
  S-Function/1 -> Demux/1
  XRC DWClear/1 -> Mux/7
  Demux/4 -> XRC Data Written/1
  XRC Data Written/1 -> Data Written/1
  DWClear/1 -> Convert3/1
  Convert3/1 -> XRC DWClear/1

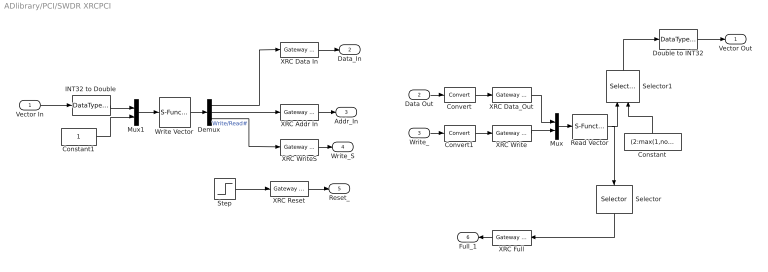
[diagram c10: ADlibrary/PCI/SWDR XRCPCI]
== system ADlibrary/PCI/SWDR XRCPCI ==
  Vector In : Inport
  Data Out : Inport  Port=2
  Write_ : Inport  Port=3
  Constant : Constant  Orientation=up  Value=(2:max(1,no_outputs)+1)-(no_outputs==0)
  Constant1 : Constant
  Convert : xbsIndex_r3/Convert  arith_type=Unsigned  n_bits=32  bin_pt=0  quantization=Truncate  overflow=Wrap  latency=0  explicit_period=on  period=1  dbl_ovrd=off  inserted_by_tool=off
  Convert1 : xbsIndex_r3/Convert  arith_type=Boolean  n_bits=1  bin_pt=0  quantization=Truncate  overflow=Wrap  latency=0  explicit_period=on  period=1  dbl_ovrd=off  inserted_by_tool=off
  Demux : Demux  Outputs=3
  Double to INT32 : DataTypeConversion  DataType=uint32
  INT32 to Double : DataTypeConversion  DataType=double
  Mux : Mux  Inputs=2
  Mux1 : Mux  Inputs=2
  Read Vector : S-Function  FunctionName=readvec_dma  Parameters=no_inputs no_outputs circuit_lag fifo_length debug
  Selector : Selector  Orientation=down
  Selector1 : Selector  Orientation=up  ElementSrc=External
  Step : Step  Before=1  After=0  SampleTime=1
  Write Vector : S-Function  FunctionName=writevec_slave  Parameters=no_inputs no_outputs circuit_lag
  XRC Addr In : xbsIndex_r3/Gateway In  arith_type=Unsigned  n_bits=22  bin_pt=0  quantization=Truncate  overflow=Wrap  period=1  timing_constraint=None  locs_specified=off  LOCs={}  needs_fixed_name=on  dbl_ovrd=off
  XRC Data In : xbsIndex_r3/Gateway In  arith_type=Unsigned  n_bits=32  bin_pt=0  quantization=Truncate  overflow=Wrap  period=1  timing_constraint=None  locs_specified=off  LOCs={}  needs_fixed_name=on  dbl_ovrd=off
  XRC Data_Out : xbsIndex_r3/Gateway Out  hdl_port=on  timing_constraint=None  locs_specified=off  LOCs={}  needs_fixed_name=on
  XRC Full : xbsIndex_r3/Gateway In  Orientation=left  arith_type=Boolean  n_bits=1  bin_pt=0  quantization=Truncate  overflow=Wrap  period=1  timing_constraint=None  locs_specified=off  LOCs={}  needs_fixed_name=on  dbl_ovrd=off
  XRC Reset : xbsIndex_r3/Gateway In  arith_type=Boolean  n_bits=1  bin_pt=0  quantization=Truncate  overflow=Wrap  period=1  timing_constraint=None  locs_specified=off  LOCs={}  needs_fixed_name=on  dbl_ovrd=off
  XRC Write : xbsIndex_r3/Gateway Out  hdl_port=on  timing_constraint=None  locs_specified=off  LOCs={}  needs_fixed_name=on
  XRC WriteS : xbsIndex_r3/Gateway In  arith_type=Boolean  n_bits=1  bin_pt=0  quantization=Truncate  overflow=Wrap  period=1  timing_constraint=None  locs_specified=off  LOCs={}  needs_fixed_name=on  dbl_ovrd=off
  Vector Out : Outport
  Data_In : Outport  Port=2
  Addr_In : Outport  Port=3
  Write_S : Outport  Port=4
  Reset_ : Outport  Port=5
  Full_1 : Outport  Orientation=left  Port=6
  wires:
  Vector In/1 -> INT32 to Double/1
  Double to INT32/1 -> Vector Out/1
  Mux/1 -> Read Vector/1
  Mux1/1 -> Write Vector/1
  INT32 to Double/1 -> Mux1/1
  XRC Data_Out/1 -> Mux/1
  XRC Write/1 -> Mux/2
  Read Vector/1 -> Selector1/1, Selector/1
  Selector1/1 -> Double to INT32/1
  Constant/1 -> Selector1/2
  Convert/1 -> XRC Data_Out/1
  Convert1/1 -> XRC Write/1
  Selector/1 -> XRC Full/1
  XRC Full/1 -> Full_1/1
  Data Out/1 -> Convert/1
  Write_/1 -> Convert1/1
  Constant1/1 -> Mux1/2
  Demux/3 -> XRC WriteS/1  "Write/Read#"
  Demux/2 -> XRC Addr In/1
  Demux/1 -> XRC Data In/1
  XRC Data In/1 -> Data_In/1
  XRC Addr In/1 -> Addr_In/1
  XRC WriteS/1 -> Write_S/1
  Write Vector/1 -> Demux/1
  Step/1 -> XRC Reset/1
  XRC Reset/1 -> Reset_/1

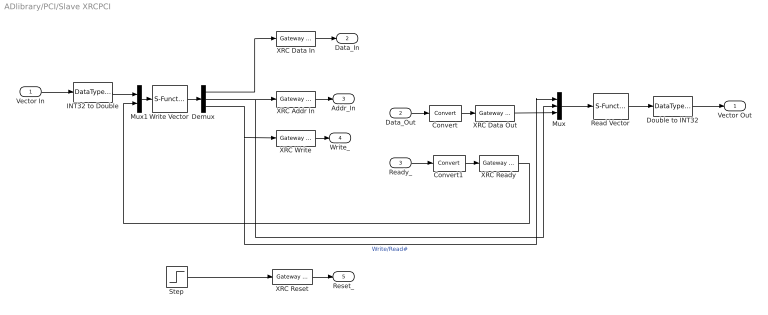
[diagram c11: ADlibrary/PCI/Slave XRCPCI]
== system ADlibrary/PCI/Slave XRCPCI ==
  Vector In : Inport
  Data_Out : Inport  Port=2
  Ready_ : Inport  Port=3
  Convert : xbsIndex_r3/Convert  arith_type=Unsigned  n_bits=32  bin_pt=0  quantization=Truncate  overflow=Wrap  latency=0  explicit_period=on  period=1  dbl_ovrd=off  inserted_by_tool=off
  Convert1 : xbsIndex_r3/Convert  arith_type=Boolean  n_bits=1  bin_pt=0  quantization=Truncate  overflow=Wrap  latency=0  explicit_period=on  period=1  dbl_ovrd=off  inserted_by_tool=off
  Demux : Demux  Outputs=3
  Double to INT32 : DataTypeConversion  DataType=uint32
  INT32 to Double : DataTypeConversion  DataType=double
  Mux : Mux  Inputs=3
  Mux1 : Mux  Inputs=2
  Read Vector : S-Function  FunctionName=readvec_slave  Parameters=no_inputs no_outputs circuit_lag decode_delay
  Step : Step  Before=1  After=0  SampleTime=1
  Write Vector : S-Function  FunctionName=writevec_slave  Parameters=no_inputs no_outputs circuit_lag
  XRC Addr In : xbsIndex_r3/Gateway In  arith_type=Unsigned  n_bits=22  bin_pt=0  quantization=Truncate  overflow=Wrap  period=1  timing_constraint=None  locs_specified=off  LOCs={}  needs_fixed_name=on  dbl_ovrd=off
  XRC Data In : xbsIndex_r3/Gateway In  arith_type=Unsigned  n_bits=32  bin_pt=0  quantization=Truncate  overflow=Wrap  period=1  timing_constraint=None  locs_specified=off  LOCs={}  needs_fixed_name=on  dbl_ovrd=off
  XRC Data Out : xbsIndex_r3/Gateway Out  hdl_port=on  timing_constraint=None  locs_specified=off  LOCs={}  needs_fixed_name=on
  XRC Ready : xbsIndex_r3/Gateway Out  hdl_port=on  timing_constraint=None  locs_specified=off  LOCs={}  needs_fixed_name=on
  XRC Reset : xbsIndex_r3/Gateway In  arith_type=Boolean  n_bits=1  bin_pt=0  quantization=Truncate  overflow=Wrap  period=1  timing_constraint=None  locs_specified=off  LOCs={}  needs_fixed_name=on  dbl_ovrd=off
  XRC Write : xbsIndex_r3/Gateway In  arith_type=Boolean  n_bits=1  bin_pt=0  quantization=Truncate  overflow=Wrap  period=1  timing_constraint=None  locs_specified=off  LOCs={}  needs_fixed_name=on  dbl_ovrd=off
  Vector Out : Outport
  Data_In : Outport  Port=2
  Addr_In : Outport  Port=3
  Write_ : Outport  Port=4
  Reset_ : Outport  Port=5
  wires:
  Mux/1 -> Read Vector/1
  Demux/3 -> Mux/1, XRC Write/1  "Write/Read#"
  Demux/2 -> Mux/2, XRC Addr In/1
  Demux/1 -> XRC Data In/1
  Write Vector/1 -> Demux/1
  Read Vector/1 -> Double to INT32/1
  XRC Ready/1 -> Mux1/2
  Mux1/1 -> Write Vector/1
  INT32 to Double/1 -> Mux1/1
  Step/1 -> XRC Reset/1
  Vector In/1 -> INT32 to Double/1
  Double to INT32/1 -> Vector Out/1
  XRC Data Out/1 -> Mux/3
  Convert/1 -> XRC Data Out/1
  Convert1/1 -> XRC Ready/1
  Data_Out/1 -> Convert/1
  Ready_/1 -> Convert1/1
  XRC Data In/1 -> Data_In/1
  XRC Addr In/1 -> Addr_In/1
  XRC Write/1 -> Write_/1
  XRC Reset/1 -> Reset_/1

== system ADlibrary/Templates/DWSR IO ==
  Vector Input : Inport
  " System Generator" : xbsIndex_r3/ System Generator  Tag=genX  xilinxfamily=Virtex2  part=xc2v3000  speed=-4  package=ff1152  synthesis_tool=XST  directory=D:/matlabR12/toolbox/xilinx/sysgen/bin  testbench=off  simulink_period=1  sysclk_period=100  trim_vbits=According to Block Masks  dbl_ovrd=According to Block Masks  core_generation=According to Block Masks  run_coregen=off  deprecated_control=off
  ADMXRC Board  Implementation : ADlibrary/Miscellaneous/ADMXRC Board  Implementation  board=<empty>  run_synth=off  make_clean=off  lvds_io_std=3.3v  clock_source=MCLK
  DWSR XRCPCI : ADlibrary/PCI/DWSR XRCPCI  AncestorBlock=ADlibrary/PCI/Slave XRCPCI  no_inputs=1  no_outputs=1  circuit_lag=1  decode_delay=0
  Vector Output : Outport
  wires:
  Vector Input/1 -> DWSR XRCPCI/1
  DWSR XRCPCI/1 -> Vector Output/1

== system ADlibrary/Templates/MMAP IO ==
  Data Input : Inport
  Addr : Inport  Port=2
  Write : Inport  Port=3
  " System Generator" : xbsIndex_r3/ System Generator  Tag=genX  xilinxfamily=Virtex2  part=xc2v3000  speed=-4  package=ff1152  synthesis_tool=XST  directory=D:/matlabR12/toolbox/xilinx/sysgen/bin  testbench=off  simulink_period=1  sysclk_period=100  trim_vbits=According to Block Masks  dbl_ovrd=According to Block Masks  core_generation=According to Block Masks  run_coregen=off  deprecated_control=off
  ADMXRC Board  Implementation : ADlibrary/Miscellaneous/ADMXRC Board  Implementation  board=<empty>  run_synth=off  make_clean=off  lvds_io_std=3.3v  clock_source=MCLK
  MMAP XRCPCI : ADlibrary/PCI/MMAP XRCPCI  AncestorBlock=ADlibrary/PCI/DWSR XRCPCI  qv132678sdfs=0
  Data Output : Outport
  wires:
  Data Input/1 -> MMAP XRCPCI/1
  Addr/1 -> MMAP XRCPCI/2
  Write/1 -> MMAP XRCPCI/3
  MMAP XRCPCI/1 -> Data Output/1

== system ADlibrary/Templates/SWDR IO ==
  Vector Input : Inport
  " System Generator" : xbsIndex_r3/ System Generator  Tag=genX  xilinxfamily=Virtex2  part=xc2v3000  speed=-4  package=ff1152  synthesis_tool=XST  directory=D:/matlabR12/toolbox/xilinx/sysgen/bin  testbench=off  simulink_period=1  sysclk_period=100  trim_vbits=According to Block Masks  dbl_ovrd=According to Block Masks  core_generation=According to Block Masks  run_coregen=off  deprecated_control=off
  ADMXRC Board  Implementation : ADlibrary/Miscellaneous/ADMXRC Board  Implementation  board=<empty>  run_synth=off  make_clean=off  lvds_io_std=3.3v  clock_source=MCLK
  SWDR XRCPCI : ADlibrary/PCI/SWDR XRCPCI  AncestorBlock=ADlibrary/PCI/ADMA XRCPCI  no_inputs=1  no_outputs=1  circuit_lag=4  fifo_length=256  debug=0
  Vector Output : Outport
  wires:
  Vector Input/1 -> SWDR XRCPCI/1
  SWDR XRCPCI/1 -> Vector Output/1

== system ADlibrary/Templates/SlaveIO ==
  Vector Input : Inport
  " System Generator" : xbsIndex_r3/ System Generator  Tag=genX  xilinxfamily=Virtex2  part=xc2v3000  speed=-4  package=ff1152  synthesis_tool=XST  directory=D:/matlabR12/toolbox/xilinx/sysgen/bin  testbench=off  simulink_period=1  sysclk_period=100  trim_vbits=According to Block Masks  dbl_ovrd=According to Block Masks  core_generation=According to Block Masks  run_coregen=off  deprecated_control=off
  ADMXRC Board  Implementation : ADlibrary/Miscellaneous/ADMXRC Board  Implementation  board=<empty>  run_synth=off  make_clean=off  lvds_io_std=3.3v  clock_source=MCLK
  Slave XRCPCI : ADlibrary/PCI/Slave XRCPCI  no_inputs=1  no_outputs=1  circuit_lag=1  decode_delay=0
  Vector Output : Outport
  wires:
  Vector Input/1 -> Slave XRCPCI/1
  Slave XRCPCI/1 -> Vector Output/1
